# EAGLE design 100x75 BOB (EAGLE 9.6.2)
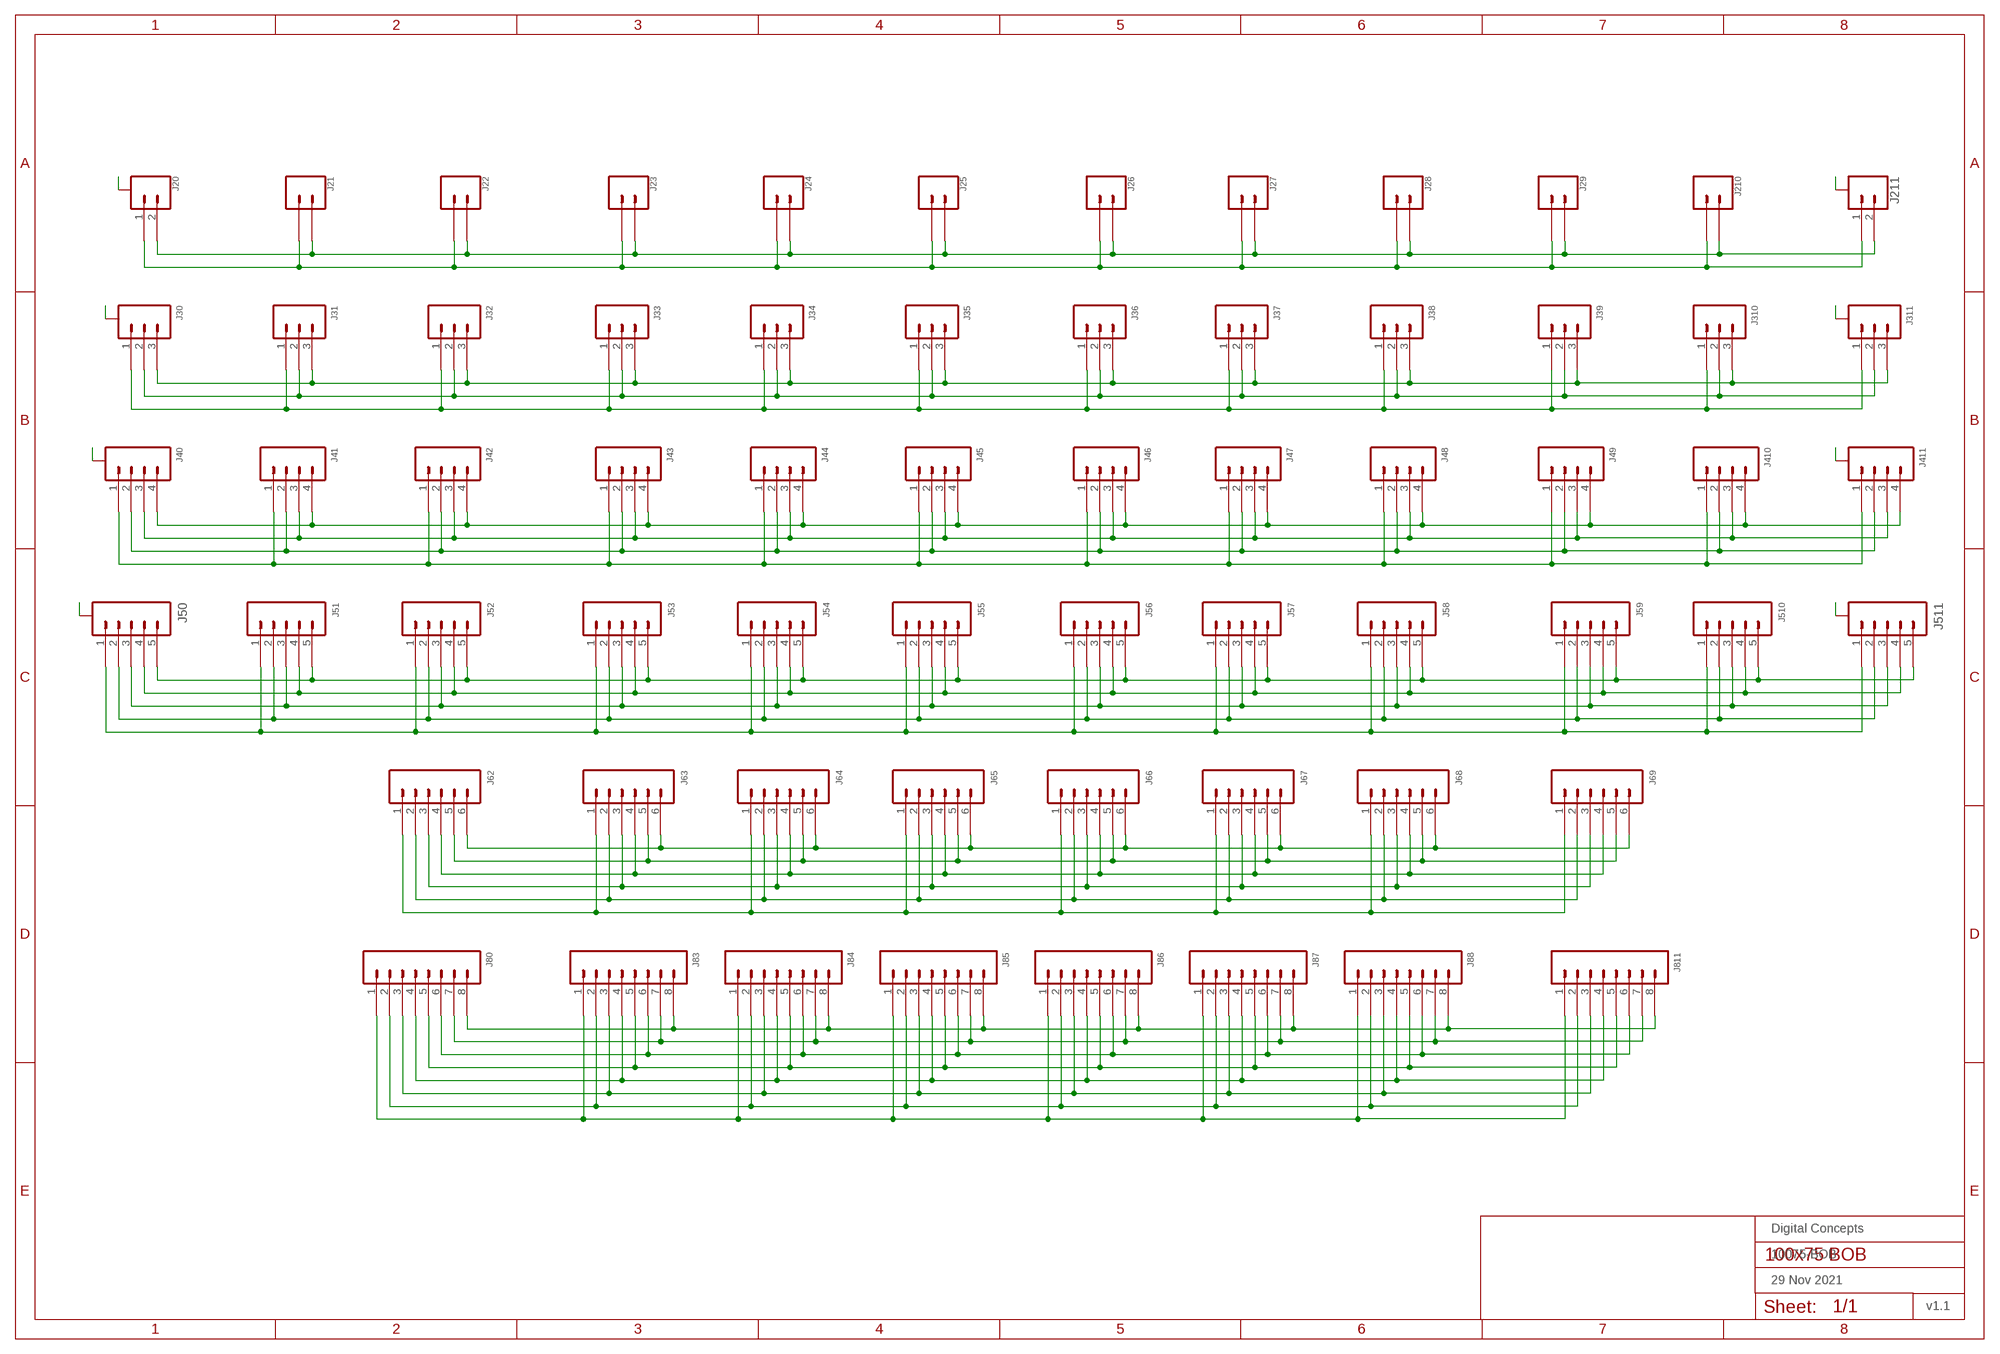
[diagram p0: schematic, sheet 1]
FRAME1 (FRAME-A3L-LOC): DATE: 29 Nov 2021; OWNER: Digital Concepts; TITLE: 10075-BOB; VERSION: v1.1

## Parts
J20  JST-SH1.0-2-SMD-VERTICAL  [JST-SH1.0-2-VERTICAL]
J21  JST-GH1.25-2-VERTICAL  [JST-GH1.25-2-VERTICAL]
J22  JST-PH2.0-2-VERTICAL  [JST-PH2.0-2-VERTICAL]
J23  HEADER-1X2-GENERIC  [CONN_02-GENERIC]
J24  HEADER-1X2-GENERIC  [CONN_02-GENERIC]
J25  HEADER-1X2-GENERIC  [CONN_02-GENERIC]
J26  HEADER-1X2-GENERIC  [CONN_02-GENERIC]
J27  HEADER-1X2-GENERIC  [CONN_02-GENERIC]
J28  HEADER-1X2-GENERIC  [CONN_02-GENERIC]
J29  JST-PH2.0-2-VERTICAL  [JST-PH2.0-2-VERTICAL]
J30  JST-SH1.0-3-SMD-VERTICAL  [JST-SH1.0-3-VERTICAL]
J31  JST-GH1.25-3-VERTICAL  [JST-GH1.25-3-VERTICAL]
J32  JST-PH2.0-3-VERTICAL  [JST-PH2.0-3-VERTICAL]
J33  HEADER-1X3-GENERIC  [CONN_03-GENERIC]
J34  HEADER-1X3-GENERIC  [CONN_03-GENERIC]
J35  HEADER-1X3-GENERIC  [CONN_03-GENERIC]
J36  HEADER-1X3-GENERIC  [CONN_03-GENERIC]
J37  HEADER-1X3-GENERIC  [CONN_03-GENERIC]
J38  HEADER-1X3-GENERIC  [CONN_03-GENERIC]
J39  JST-PH2.0-3-VERTICAL  [JST-PH2.0-3-VERTICAL]
J40  JST-SH1.0-4-SMD-VERTICAL  [JST-SH1.0-4-VERTICAL]
J41  JST-GH1.25-4-VERTICAL  [JST-GH1.25-4-VERTICAL]
J42  JST-PH2.0-4-VERTICAL  [JST-PH2.0-4-VERTICAL]
J43  HEADER-1X4-GENERIC  [CONN_04-GENERIC]
J44  HEADER-1X4-GENERIC  [CONN_04-GENERIC]
J45  HEADER-1X4-GENERIC  [CONN_04-GENERIC]
J46  HEADER-1X4-GENERIC  [CONN_04-GENERIC]
J47  HEADER-1X4-GENERIC  [CONN_04-GENERIC]
J48  HEADER-1X4-GENERIC  [CONN_04-GENERIC]
J49  JST-PH2.0-4-VERTICAL  [JST-PH2.0-4-VERTICAL]
J50  JST-SH1.0-5-SMD-VERTICAL  [JST-SH1.0-5-VERTICAL]
J51  JST-GH1.25-5-VERTICAL  [JST-GH1.25-5-VERTICAL]
J52  JST-PH2.0-5-VERTICAL  [JST-PH2.0-5-VERTICAL]
J53  HEADER-1X5-GENERIC  [CONN_05-GENERIC]
J54  HEADER-1X5-GENERIC  [CONN_05-GENERIC]
J55  HEADER-1X5-GENERIC  [CONN_05-GENERIC]
J56  HEADER-1X5-GENERIC  [CONN_05-GENERIC]
J57  HEADER-1X5-GENERIC  [CONN_05-GENERIC]
J58  HEADER-1X5-GENERIC  [CONN_05-GENERIC]
J59  JST-PH2.0-5-VERTICAL  [JST-PH2.0-5-VERTICAL]
J62  RJ11-6P6C-VERTICAL  [RJ11-6-VERTICAL]
J63  HEADER-1X6-GENERIC  [CONN_06-GENERIC]
J64  HEADER-1X6-GENERIC  [CONN_06-GENERIC]
J65  HEADER-1X6-GENERIC  [CONN_06-GENERIC]
J66  HEADER-1X6-GENERIC  [CONN_06-GENERIC]
J67  HEADER-1X6-GENERIC  [CONN_06-GENERIC]
J68  HEADER-1X6-GENERIC  [CONN_06-GENERIC]
J69  RJ11-6P6C-VERTICAL  [RJ11-6-VERTICAL]
J80  RJ45-8P8C-VERTICAL-MK2  [RJ45-VERTICAL-MK2]
J83  HEADER-1X8-GENERIC  [CONN_08-GENERIC]
J84  HEADER-1X8-GENERIC  [CONN_08-GENERIC]
J85  HEADER-1X8-GENERIC  [CONN_08-GENERIC]
J86  HEADER-1X8-GENERIC  [CONN_08-GENERIC]
J87  HEADER-1X8-GENERIC  [CONN_08-GENERIC]
J88  HEADER-1X8-GENERIC  [CONN_08-GENERIC]
J210  JST-GH1.25-2-VERTICAL  [JST-GH1.25-2-VERTICAL]
J211  JST-SH1.0-2-SMD-VERTICAL  [JST-SH1.0-2-VERTICAL]
J310  JST-GH1.25-3-VERTICAL  [JST-GH1.25-3-VERTICAL]
J311  JST-SH1.0-3-SMD-VERTICAL  [JST-SH1.0-3-VERTICAL]
J410  JST-GH1.25-4-VERTICAL  [JST-GH1.25-4-VERTICAL]
J411  JST-SH1.0-4-SMD-VERTICAL  [JST-SH1.0-4-VERTICAL]
J510  JST-GH1.25-5-VERTICAL  [JST-GH1.25-5-VERTICAL]
J511  JST-SH1.0-5-SMD-VERTICAL  [JST-SH1.0-5-VERTICAL]
J811  RJ45-8P8C-VERTICAL-MK2  [RJ45-VERTICAL-MK2]

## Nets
A: J20.A@1(A) J20.A@2(A) J30.A@1(A) J30.A@3(A) J40.A@1(A) J40.A@4(A) J50.A@1(A) J50.A@5(A) J211.A@1(A) J211.A@2(A) J311.A@1(A) J311.A@3(A) J411.A@1(A) J411.A@4(A) J511.A@1(A) J511.A@5(A)
N$1: J20.1 J21.1 J22.1 J23.1 J24.1 J25.1 J26.1 J27.1 J28.1 J29.1 J210.1 J211.1
N$2: J30.3 J31.3 J32.3 J33.3 J34.3 J35.3 J36.3 J37.3 J38.3 J39.3 J310.3 J311.3
N$3: J30.2 J31.2 J32.2 J33.2 J34.2 J35.2 J36.2 J37.2 J38.2 J39.2 J310.2 J311.2
N$4: J30.1 J31.1 J32.1 J33.1 J34.1 J35.1 J36.1 J37.1 J38.1 J39.1 J310.1 J311.1
N$5: J80.8 J83.8 J84.8 J85.8 J86.8 J87.8 J88.8 J811.8
N$6: J80.7 J83.7 J84.7 J85.7 J86.7 J87.7 J88.7 J811.7
N$7: J20.2 J21.2 J22.2 J23.2 J24.2 J25.2 J26.2 J27.2 J28.2 J29.2 J210.2 J211.2
N$8: J80.6 J83.6 J84.6 J85.6 J86.6 J87.6 J88.6 J811.6
N$9: J80.5 J83.5 J84.5 J85.5 J86.5 J87.5 J88.5 J811.5
N$10: J80.4 J83.4 J84.4 J85.4 J86.4 J87.4 J88.4 J811.4
N$11: J80.3 J83.3 J84.3 J85.3 J86.3 J87.3 J88.3 J811.3
N$12: J80.2 J83.2 J84.2 J85.2 J86.2 J87.2 J88.2 J811.2
N$13: J80.1 J83.1 J84.1 J85.1 J86.1 J87.1 J88.1 J811.1
N$14: J62.6 J63.6 J64.6 J65.6 J66.6 J67.6 J68.6 J69.6
N$15: J62.5 J63.5 J64.5 J65.5 J66.5 J67.5 J68.5 J69.5
N$16: J62.4 J63.4 J64.4 J65.4 J66.4 J67.4 J68.4 J69.4
N$17: J62.3 J63.3 J64.3 J65.3 J66.3 J67.3 J68.3 J69.3
N$18: J62.2 J63.2 J64.2 J65.2 J66.2 J67.2 J68.2 J69.2
N$19: J62.1 J63.1 J64.1 J65.1 J66.1 J67.1 J68.1 J69.1
N$20: J40.1 J41.1 J42.1 J43.1 J44.1 J45.1 J46.1 J47.1 J48.1 J49.1 J410.1 J411.1
N$21: J40.2 J41.2 J42.2 J43.2 J44.2 J45.2 J46.2 J47.2 J48.2 J49.2 J410.2 J411.2
N$22: J40.3 J41.3 J42.3 J43.3 J44.3 J45.3 J46.3 J47.3 J48.3 J49.3 J410.3 J411.3
N$23: J40.4 J41.4 J42.4 J43.4 J44.4 J45.4 J46.4 J47.4 J48.4 J49.4 J410.4 J411.4
N$25: J50.4 J51.4 J52.4 J53.4 J54.4 J55.4 J56.4 J57.4 J58.4 J59.4 J510.4 J511.4
N$26: J50.3 J51.3 J52.3 J53.3 J54.3 J55.3 J56.3 J57.3 J58.3 J59.3 J510.3 J511.3
N$27: J50.2 J51.2 J52.2 J53.2 J54.2 J55.2 J56.2 J57.2 J58.2 J59.2 J510.2 J511.2
N$28: J50.1 J51.1 J52.1 J53.1 J54.1 J55.1 J56.1 J57.1 J58.1 J59.1 J510.1 J511.1
N$30: J50.5 J51.5 J52.5 J53.5 J54.5 J55.5 J56.5 J57.5 J58.5 J59.5 J510.5 J511.5

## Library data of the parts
J20 J211 = digitalconcepts:JST-SH1.0-2-SMD-VERTICAL: JST SH1.0 2P SMD Vertical Connector
J21 J210 = digitalconcepts:JST-GH1.25-2-VERTICAL: JST GH1.25 2P PTH Connector
J22 J29 = digitalconcepts:JST-PH2.0-2-VERTICAL: PH2.0 2P Vertical Connector
J23-J28 = digitalconcepts:HEADER-1X2-GENERIC: Single Row 2-Pin Header
J30 J311 = digitalconcepts:JST-SH1.0-3-SMD-VERTICAL: JST SH1.0 3P SMD Vertical Connector
J31 J310 = digitalconcepts:JST-GH1.25-3-VERTICAL: SH1.25 3P Male PTH Connector
J32 J39 = digitalconcepts:JST-PH2.0-3-VERTICAL: PH2.0 3P Vertical Connector
J33-J38 = digitalconcepts:HEADER-1X3-GENERIC: Single Row 3-Pin Header
J40 J411 = digitalconcepts:JST-SH1.0-4-SMD-VERTICAL: JST SH1.0 SMD 4P vertical connector
J41 J410 = digitalconcepts:JST-GH1.25-4-VERTICAL: SH1.25 4P Male PTH Connector
J42 J49 = digitalconcepts:JST-PH2.0-4-VERTICAL: PH2.0 4P Vertical Connector
J43-J48 = digitalconcepts:HEADER-1X4-GENERIC: Single Row 4-Pin Header
J50 J511 = digitalconcepts:JST-SH1.0-5-SMD-VERTICAL: JST SH1.0 5P SMD Vertical Connector
J51 J510 = digitalconcepts:JST-GH1.25-5-VERTICAL: SH1.25 5P Male PTH Connector
J52 J59 = digitalconcepts:JST-PH2.0-5-VERTICAL: PH2.0 5P Vertical Connector
J53-J58 = digitalconcepts:HEADER-1X5-GENERIC: Single Row 5-Pin Header
J62 J69 = digitalconcepts:RJ11-6P6C-VERTICAL: RJ11-6P6C-Vertical PCB Socket
J63-J68 = digitalconcepts:HEADER-1X6-GENERIC: Single Row 6-Pin Header
J80 J811 = digitalconcepts:RJ45-8P8C-VERTICAL-MK2: RJ45-8P8C-Vertical PCB Socket
J83-J88 = digitalconcepts:HEADER-1X8-GENERIC: Single Row 8-Pin Header

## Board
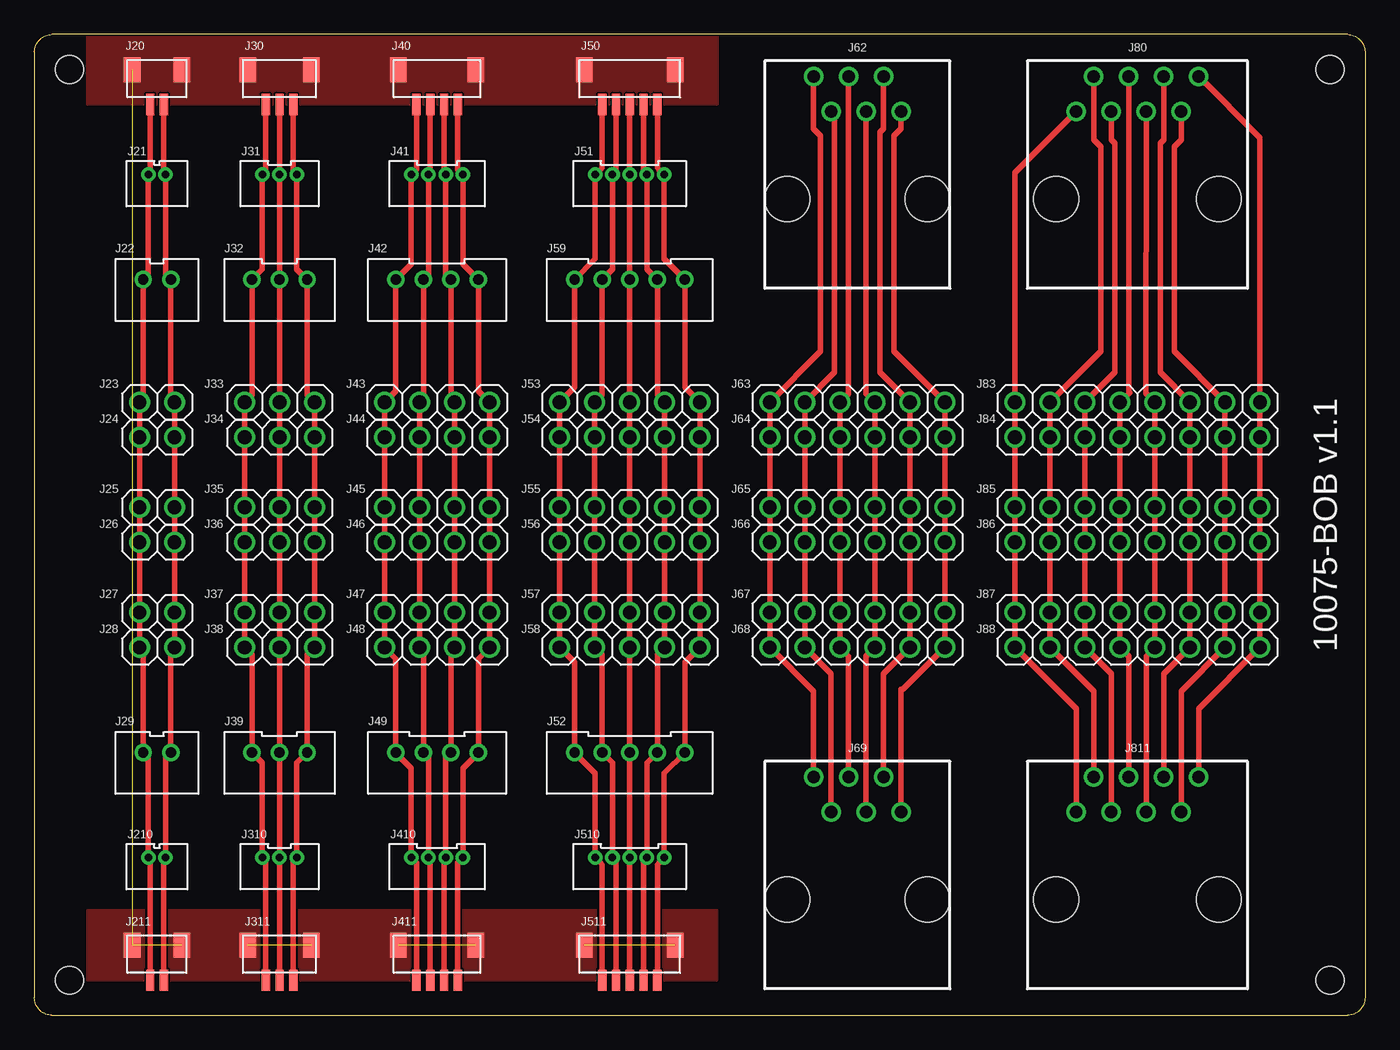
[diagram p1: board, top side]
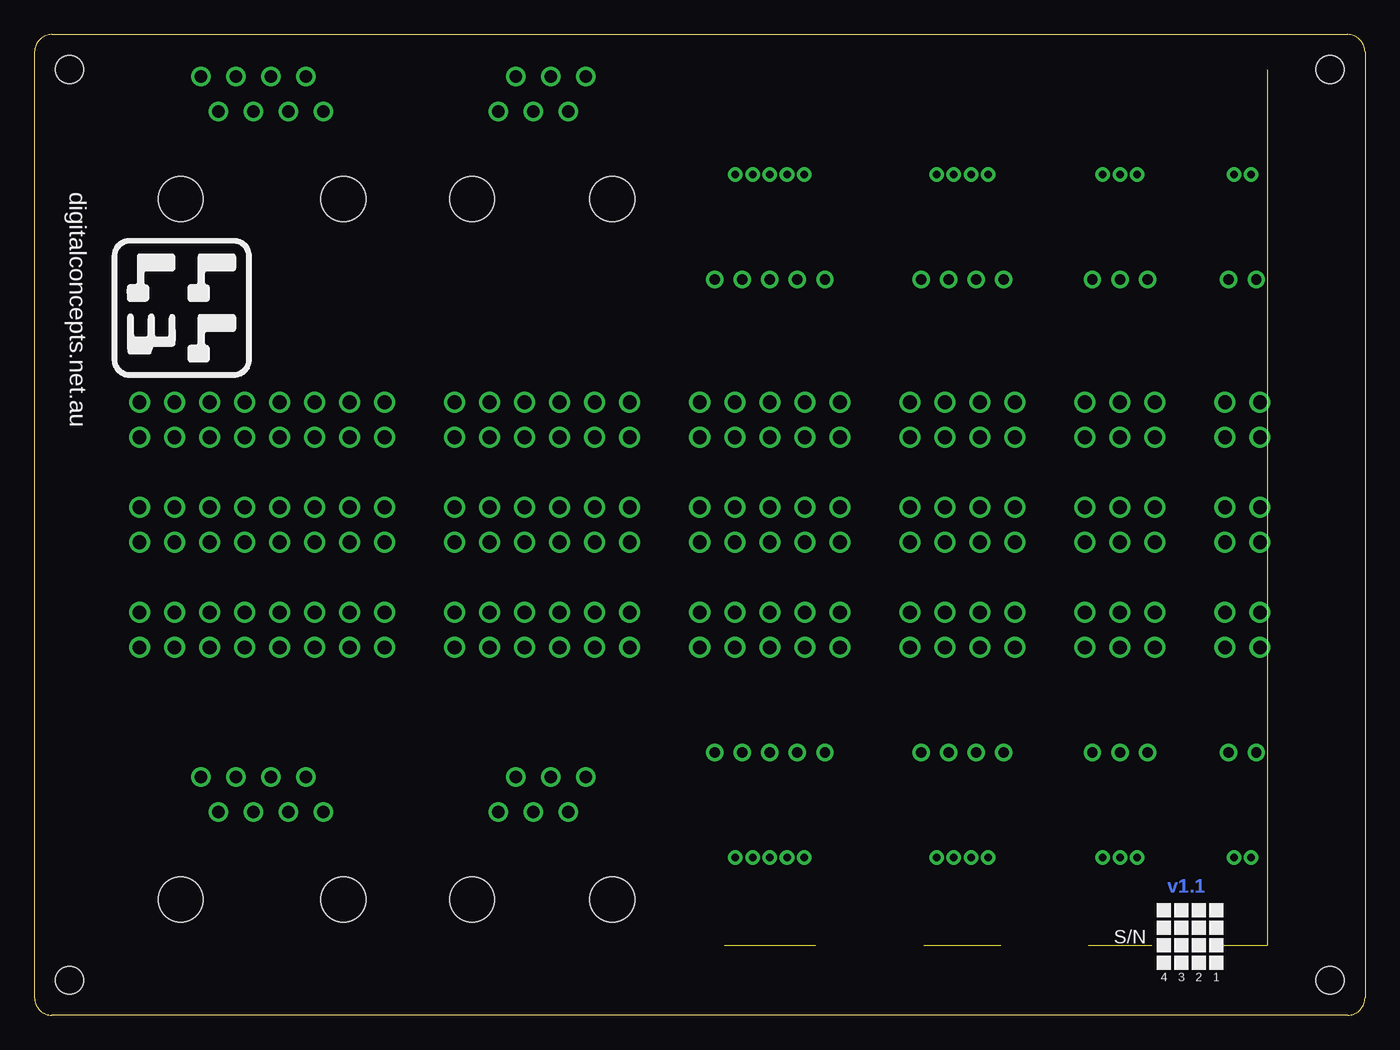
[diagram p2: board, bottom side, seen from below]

Size 96.52 x 71.12 mm. Coordinates in mm from the lower left corner, seen from the top.
Outline: 95.25,71.12 arc-90 96.52,69.85 96.52,1.27 arc-90 95.25,0 1.27,0 arc-90 0,1.27 0,69.85 arc-90 1.27,71.12 95.25,71.12
Copper layers (1*16): Top 0.035mm / dielectric 1.5mm / Bottom 0.035mm
Design rules "default *": minimum track width 6mil, minimum drill 0.35mm, track to track 6mil, track to pad 6mil, pad to pad 6mil, via to via 6mil, smd to smd 6mil, copper to edge 6mil, drill to drill 6mil, minimum pad ring 10mil, minimum via ring 8mil, stop-mask expansion 4mil, vias tented up to drill 0mil, thermal gap 0mil
Holes 2.03 mm at 2.54,68.58 2.54,2.54 93.98,2.54 93.98,68.58

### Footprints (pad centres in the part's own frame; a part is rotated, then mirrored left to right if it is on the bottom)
JST-SH1.0-2-VERTICAL = smd 0.6 x 1.55: 1 -0.5,-2.54; 2 0.5,-2.54 | smd 1.2 x 1.8: A@1 -1.8,-0.015; A@2 1.8,-0.015
JST-GH1.25-2-VERTICAL = drill 0.55 pad 1.016: 1 -0.625,0; 2 0.625,0
JST-PH2.0-2-VERTICAL = drill 0.75: 1 -1,0; 2 1,0
CONN_02-GENERIC = drill 1 pad 1.524: 1 0,0; 2 2.54,0
JST-SH1.0-3-VERTICAL = smd 0.6 x 1.55: 1 -1,-2.54; 2 0,-2.54; 3 1,-2.54 | smd 1.2 x 1.8: A@1 -2.3,-0.015; A@3 2.3,-0.015
JST-GH1.25-3-VERTICAL = drill 0.55 pad 1.016: 1 -1.25,0; 2 0,0; 3 1.25,0
JST-PH2.0-3-VERTICAL = drill 0.75: 1 -2,0; 2 0,0; 3 2,0
CONN_03-GENERIC = drill 1 pad 1.524: 1 0,0; 2 2.54,0; 3 5.08,0
JST-SH1.0-4-VERTICAL = smd 0.6 x 1.55: 1 -1.5,-2.54; 2 -0.5,-2.54; 3 0.5,-2.54; 4 1.5,-2.54 | smd 1.2 x 1.8: A@1 -2.8,-0.015; A@4 2.8,-0.015
JST-GH1.25-4-VERTICAL = drill 0.55 pad 1.016: 1 -1.875,0; 2 -0.625,0; 3 0.625,0; 4 1.875,0
JST-PH2.0-4-VERTICAL = drill 0.75: 1 -3,0; 2 -1,0; 3 1,0; 4 3,0
CONN_04-GENERIC = drill 1 pad 1.524: 1 0,0; 2 2.54,0; 3 5.08,0; 4 7.62,0
JST-SH1.0-5-VERTICAL = smd 0.6 x 1.55: 1 -2,-2.54; 2 -1,-2.54; 3 0,-2.54; 4 1,-2.54; 5 2,-2.54 | smd 1.2 x 1.8: A@1 -3.3,-0.015; A@5 3.3,-0.015
JST-GH1.25-5-VERTICAL = drill 0.55 pad 1.016: 1 -2.5,0; 2 -1.25,0; 3 0,0; 4 1.25,0; 5 2.5,0
JST-PH2.0-5-VERTICAL = drill 0.75: 1 -4,0; 2 -2,0; 3 0,0; 4 2,0; 5 4,0
CONN_05-GENERIC = drill 1 pad 1.524: 1 0,0; 2 2.54,0; 3 5.08,0; 4 7.62,0; 5 10.16,0
RJ11-6-VERTICAL = drill 0.9: 1 -3.175,7.12; 2 -1.905,4.58; 3 -0.635,7.12; 4 0.635,4.58; 5 1.905,7.12; 6 3.175,4.58 | hole 3.25: -5.08,-1.77; 5.08,-1.77
CONN_06-GENERIC = drill 1 pad 1.524: 1 0,0; 2 2.54,0; 3 5.08,0; 4 7.62,0; 5 10.16,0; 6 12.7,0
RJ45-VERTICAL-MK2 = drill 0.9: 1 -4.445,4.58; 2 -3.175,7.12; 3 -1.905,4.58; 4 -0.635,7.12; 5 0.635,4.58; 6 1.905,7.12; 7 3.175,4.58; 8 4.445,7.12 | hole 3.25: -5.9,-1.77; 5.9,-1.77
CONN_08-GENERIC = drill 1 pad 1.524: 1 0,0; 2 2.54,0; 3 5.08,0; 4 7.62,0; 5 10.16,0; 6 12.7,0; 7 15.24,0; 8 17.78,0

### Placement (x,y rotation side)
J20  8.89,68.58 0 top
J21  8.89,60.96 0 top
J22  8.89,53.34 0 top
J23  7.62,44.45 0 top
J24  7.62,41.91 0 top
J25  7.62,36.83 0 top
J26  7.62,34.29 0 top
J27  7.62,29.21 0 top
J28  7.62,26.67 0 top
J29  8.89,19.05 0 top
J30  17.78,68.58 0 top
J31  17.78,60.96 0 top
J32  17.78,53.34 0 top
J33  15.24,44.45 0 top
J34  15.24,41.91 0 top
J35  15.24,36.83 0 top
J36  15.24,34.29 0 top
J37  15.24,29.21 0 top
J38  15.24,26.67 0 top
J39  17.78,19.05 0 top
J40  29.21,68.58 0 top
J41  29.21,60.96 0 top
J42  29.21,53.34 0 top
J43  25.4,44.45 0 top
J44  25.4,41.91 0 top
J45  25.4,36.83 0 top
J46  25.4,34.29 0 top
J47  25.4,29.21 0 top
J48  25.4,26.67 0 top
J49  29.21,19.05 0 top
J50  43.18,68.58 0 top
J51  43.18,60.96 0 top
J52  43.18,19.05 0 top
J53  38.1,44.45 0 top
J54  38.1,41.91 0 top
J55  38.1,36.83 0 top
J56  38.1,34.29 0 top
J57  38.1,29.21 0 top
J58  38.1,26.67 0 top
J59  43.18,53.34 0 top
J62  59.69,60.96 0 top
J63  53.34,44.45 0 top
J64  53.34,41.91 0 top
J65  53.34,36.83 0 top
J66  53.34,34.29 0 top
J67  53.34,29.21 0 top
J68  53.34,26.67 0 top
J69  59.69,10.16 0 top
J80  80.01,60.96 0 top
J83  71.12,44.45 0 top
J84  71.12,41.91 0 top
J85  71.12,36.83 0 top
J86  71.12,34.29 0 top
J87  71.12,29.21 0 top
J88  71.12,26.67 0 top
J210  8.89,11.43 0 top
J211  8.89,5.08 0 top
J310  17.78,11.43 0 top
J311  17.78,5.08 0 top
J410  29.21,11.43 0 top
J411  29.21,5.08 0 top
J510  43.18,11.43 0 top
J511  43.18,5.08 0 top
J811  80.01,10.16 0 top

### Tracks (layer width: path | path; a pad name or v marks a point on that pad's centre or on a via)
A  (5 unrouted)
  pour Top: 3.81,71.12 49.53,71.12 49.53,66.04 3.81,66.04
  pour Top: 3.81,2.54 49.53,2.54 49.53,7.62 3.81,7.62
N$1
  Top 0.406: J20.1 8.39,61.09 J21.1 8.27,53.72 J22.1 7.89,44.72 J23.1 J24.1 J25.1 J26.1 J27.1 J28.1 7.89,26.4 J29.1 8.27,18.68 J210.1 8.39,11.3 J211.1
N$2
  Top 0.406: J30.3 18.78,61.21 J31.3 19.03,54.09 J32.3 19.78,44.99 J33.3 J34.3 J35.3 J36.3 J37.3 J38.3 19.78,26.13 J39.3 19.03,18.3 J310.3 18.78,11.18 J311.3
N$3
  Top 0.406: J30.2 J31.2 J32.2 J33.2 J34.2 J35.2 J36.2 J37.2 J38.2 J39.2 J310.2 J311.2
N$4
  Top 0.406: J30.1 16.78,61.21 J31.1 16.53,54.09 J32.1 15.78,44.99 J33.1 J34.1 J35.1 J36.1 J37.1 J38.1 15.78,26.13 J39.1 16.51,18.32 16.51,11.45 J310.1 16.78,11.18 J311.1
N$5
  Top 0.406: J80.8 88.9,63.63 J83.8 J84.8 J85.8 J86.8 J87.8 J88.8 84.45,22.23 J811.8
N$6
  Top 0.406: J80.7 83.19,63.5 82.68,62.99 82.68,48.13 J83.7 J84.7 J85.7 J86.7 J87.7 J88.7 83.19,23.5 J811.7
N$7
  Top 0.406: J20.2 9.39,61.09 J21.2 9.52,53.72 J22.2 9.89,44.72 J23.2 J24.2 J25.2 J26.2 J27.2 J28.2 9.89,26.4 J29.2 9.52,18.68 J210.2 9.39,11.3 J211.2
N$8
  Top 0.406: J80.6 81.92,63.5 81.66,63.25 81.66,46.61 J83.6 J84.6 J85.6 J86.6 J87.6 J88.6 81.92,24.77 J811.6
N$9
  Top 0.406: J80.5 80.64,45.09 J83.5 J84.5 J85.5 J86.5 J87.5 J88.5 80.64,26.04 J811.5
N$10
  Top 0.406: J80.4 79.38,45.22 79.44,45.15 J83.4 J84.4 J85.4 J86.4 J87.4 J88.4 79.38,26.04 J811.4
N$11
  Top 0.406: J80.3 78.11,63.5 78.36,63.25 78.36,46.61 J83.3 J84.3 J85.3 J86.3 J87.3 J88.3 78.11,24.77 J811.3
N$12
  Top 0.406: J80.2 76.83,63.5 77.34,62.99 77.34,48.13 J83.2 J84.2 J85.2 J86.2 J87.2 J88.2 76.83,23.5 J811.2
N$13
  Top 0.406: J80.1 71.12,61.09 J83.1 J84.1 J85.1 J86.1 J87.1 J88.1 75.56,22.23 J811.1
N$14
  Top 0.406: J62.6 62.87,64.27 62.36,63.76 62.36,48.13 J63.6 J64.6 J65.6 J66.6 J67.6 J68.6 63,23.63 62.87,23.63 J69.6
N$15
  Top 0.406: J62.5 61.59,64.27 61.34,64.02 61.34,46.61 J63.5 J64.5 J65.5 J66.5 J67.5 J68.5 61.59,24.77 J69.5
N$16
  Top 0.406: J62.4 60.33,45.09 J63.4 J64.4 J65.4 J66.4 J67.4 J68.4 60.33,26.04 J69.4
N$17
  Top 0.406: J62.3 59.05,45.09 J63.3 J64.3 J65.3 J66.3 J67.3 J68.3 59.05,26.04 J69.3
N$18
  Top 0.406: J62.2 58.04,65.29 58.04,46.61 J63.2 J64.2 J65.2 J66.2 J67.2 J68.2 57.78,24.77 J69.2
N$19
  Top 0.406: J62.1 56.52,64.27 57.02,63.76 57.02,48.13 J63.1 J64.1 J65.1 J66.1 J67.1 J68.1 56.52,23.5 J69.1
N$20
  Top 0.406: J40.1 27.71,61.34 27.7,61.33 J41.1 27.34,54.47 J42.1 26.21,45.26 J43.1 J44.1 J45.1 J46.1 J47.1 J48.1 26.21,25.86 J49.1 27.34,17.93 J410.1 27.7,11.06 27.71,11.05 J411.1
N$21
  Top 0.406: J40.2 28.71,61.09 J41.2 28.59,53.72 J42.2 28.21,44.72 J43.2 J44.2 J45.2 J46.2 J47.2 J48.2 28.21,26.4 J49.2 28.59,18.68 J410.2 28.71,11.3 J411.2
N$22
  Top 0.406: J40.3 29.71,61.09 J41.3 29.84,53.72 J42.3 30.21,44.72 J43.3 J44.3 J45.3 J46.3 J47.3 J48.3 30.21,26.4 J49.3 29.84,18.68 J410.3 29.71,11.3 J411.3
N$23
  Top 0.406: J40.4 30.71,61.34 30.72,61.33 J41.4 31.09,54.47 J42.4 32.21,45.26 J43.4 J44.4 J45.4 J46.4 J47.4 J48.4 32.21,25.86 J49.4 31.09,17.93 J410.4 30.72,11.06 30.71,11.05 J411.4
N$25
  Top 0.406: J50.4 44.18,61.21 J51.4 44.43,54.09 J59.4 45.18,44.99 J53.4 J54.4 J55.4 J56.4 J57.4 J58.4 45.18,26.13 J52.4 44.43,18.3 J510.4 44.18,11.18 J511.4
N$26
  Top 0.406: J50.3 J51.3 J59.3 J53.3 J54.3 J55.3 J56.3 J57.3 J58.3 J52.3 J510.3 J511.3
N$27
  Top 0.406: J50.2 42.18,61.21 J51.2 41.93,54.09 J59.2 41.18,44.99 J53.2 J54.2 J55.2 J56.2 J57.2 J58.2 41.18,26.13 J52.2 41.93,18.3 J510.2 42.18,11.18 J511.2
N$28
  Top 0.406: J50.1 41.18,61.46 41.05,61.33 J51.1 40.68,54.84 J59.1 39.18,45.53 J53.1 J54.1 J55.1 J56.1 J57.1 J58.1 39.18,25.59 J52.1 40.68,17.55 J510.1 41.05,11.06 41.18,10.93 J511.1
N$30
  Top 0.406: J50.5 45.18,61.46 45.31,61.33 J51.5 45.68,54.84 J59.5 47.18,45.53 J53.5 J54.5 J55.5 J56.5 J57.5 J58.5 47.18,25.59 J52.5 45.68,17.55 J510.5 45.31,11.06 45.18,10.93 J511.5

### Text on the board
Bottom: v1.1
tPlace: 10075-BOB v1.1
bPlace: digitalconcepts.net.au | S/N | 1 | 2 | 3 | 4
